(* Logix 5000 AddOnInstructionDefinition export I_1769scOF4IH; software revision 18.02 *)

TYPE STRING_32 :   // string type
STRUCT
   LEN : DINT;
   DATA : SINT[32];
END_STRUCT
END_TYPE

TYPE STRING_8 :   // string type
STRUCT
   LEN : DINT;
   DATA : SINT[8];
END_STRUCT
END_TYPE

TYPE P_EUTable :
STRUCT
   Code : DINT;   // Engineering Units Code Number
   Desc : STRING_8;   // Engineering Units Text
END_STRUCT
END_TYPE

TYPE HART_ChanData :   // Analog and HART Channel Data for one channel / device
STRUCT
   ModSts : SINT;   // I/O Module Status
   ChanSts : SINT;   // HART I/O Channel Status
   HARTSts : SINT;   // HART Device / Communication Status
   Initializing : BOOL;
   CommFail : BOOL;
   CurFault : BOOL;
   PassThruMSGAvail : BOOL;
   DataUpdateAvail : BOOL;
   BrokenWire : BOOL;
   StsUpdateAvail : BOOL;
   DeviceFault : BOOL;
   HARTCommErr : SINT;   // HART Communication Error Bits
   HARTCommErr0 : BOOL;
   BufferOverflow : BOOL;
   HARTCommErr2 : BOOL;
   ChecksumErr : BOOL;
   FramingErr : BOOL;
   OverrunErr : BOOL;
   ParityErr : BOOL;
   HasHARTCommErr : BOOL;
   HARTRespCode : SINT;   // HART Response Code
   HARTFieldDevSts : SINT;   // HART Field Device Status
   PVOutOfLimits : BOOL;
   VarOutOfLimits : BOOL;
   LoopCurSaturated : BOOL;
   LoopCurFixed : BOOL;
   Code48StsAvail : BOOL;
   ColdStart : BOOL;
   CfgChanged : BOOL;
   Malfunction : BOOL;
   HARTExtSts : SINT;   // HART Extended Status
   MaintReqd : BOOL;
   DeviceAlert : BOOL;
   PowerFail : BOOL;
   CalFault : BOOL;
   AV : REAL;   // Analog Value
   AVRawMin : REAL;   // Analog Signal Raw Range Minimum (here because it's not in DevInfo)
   AVRawMax : REAL;   // Analog Signal Raw Range Maximum (here because it's not in DevInfo)
   PV : REAL;   // HART Primary Variable
   SV : REAL;   // HART Secondary Variable
   TV : REAL;   // HART Tertiary Variable
   FV : REAL;   // HART Fourth Variable
   PVStatus : SINT;   // HART Primary Variable Status
   SVStatus : SINT;   // HART Secondary Variable Status
   TVStatus : SINT;   // HART Tertiary Variable Status
   FVStatus : SINT;   // HART Fourth Variable Status
   AVEU : STRING_8;   // Text for HART Range (Analog Value) Engineering Units
   PVEU : STRING_8;   // Text for HART PV Engineering Units
   SVEU : STRING_8;   // Text for HART SV Engineering Units
   TVEU : STRING_8;   // Text for HART TV Engineering Units
   FVEU : STRING_8;   // Text for HART FV Engineering Units
   Diag : SINT[28];   // Channel Diagnostic bit array (from HART Code 48 message)
   DevInfo : HART_DevInfo;   // HART Device Information
   Cfg_AutoUpdDevInfo : BOOL;   // 1=automatically update device info, 0=no auto update
   Cfg_ManUpdDevInfo : BOOL;   // 1=allow manual device info update request, 0=disallow
   MCmd_UpdDevInfo : BOOL;   // Maintenance Command to request update of device info
END_STRUCT
END_TYPE

TYPE STRING_16 :   // string type
STRUCT
   LEN : DINT;
   DATA : SINT[16];
END_STRUCT
END_TYPE

TYPE HART_DevInfo :   // HART Device Information for one channel / device
STRUCT
   CmdSts : SINT;   // HART Command Status Success=0
   MfrID : SINT;   // Manufacturer ID
   DevType : SINT;   // Device Type
   Preamble : SINT;   // HART Preamble
   UnivCmdCode : SINT;   // Universal Command Code
   XducerSpecRev : SINT;   // Transducer Specification Revision
   SwRev : SINT;   // Software Revision Number
   HwRev : SINT;   // Hardware Revision Number
   HARTFlags : SINT;   // HART Flags
   pad9 : SINT;
   MfrID_16 : INT;   // 16-bit Manufacturer ID
   DevID : DINT;   // Device ID Number (serial number)
   Tag : STRING_8;   // Tag String
   Desc : STRING_16;   // Descriptor String
   DateDay : SINT;   // Device Revision Date: Day of the Month
   DateMonth : SINT;   // Device Revision Date: Month of the Year
   DateYear : INT;   // Device Revision Date: Year
   FinalAssyNum : DINT;   // Final Assembly Number
   Message : STRING_32;   // Message String
   PVCode : SINT;   // Primary Variable Identifier
   SVCode : SINT;   // Secondary Variable Identifier
   TVCode : SINT;   // Third Variable Identifier
   FVCode : SINT;   // Fourth Variable Identifier
   PVUnits : SINT;   // Primary Variable Units of Measure (enum)
   SVUnits : SINT;   // Secondary Variable Units of Measure (enum)
   TVUnits : SINT;   // Third Variable Units of Measure (enum)
   FVUnits : SINT;   // Fourth Variable Units of Measure (enum)
   XferFunc : SINT;   // Transfer Function
   RangeUnits : SINT;   // Analog Value Range Units of Measure
   ExpDevType : INT;   // Expanded Device Type Code
   AVRangeMin : REAL;   // Analog Value in Engineering Units at 4.00 mADC
   AVRangeMax : REAL;   // Analog Value in Engineering Units at 20.00 mADC
   DampVal : REAL;   // Damping Value
   WriteProtCode : SINT;   // Write Protect Code
   pad117 : SINT;
   PrivLblMfr : INT;   // Private Label Manufacturer ID
END_STRUCT
END_TYPE

ADD_ON_INSTRUCTION I_1769scOF4IH   (* revision 3.5 01 Release, vendor Rockwell Automation *)
// Spectrum Controls 1769sc-OF4IH
// HART Isolated AO Module
// Revision note:
// See V3.5-xx Release Notes for details. New Instruction for V3.5 of Library of Premier Integration Objects.
// Help:
// Copyright © Rockwell Automation, Inc.  All Rights Reserved.
// This instruction provides 4 analog outputs for one 1769sc-OF4IH
// HART Isolated Analog output module.  It reads the input and
// configuration assemblies from the module and copies the data into
// individual structures for each of the four output channels. The
// instruction also uses a MSG instruction to read updated Device
// Information (DevInfo) for each channel.  These structures are then
// used by the P_AOutHART instruction to provide channel data,
// device configuration and diagnostic information for each individual
// HART device.
VAR_IN_OUT
   Ref_Inp : SC:1769sc_OF4IH:I:0; {required}   // HART Module Input assembly for the 1769sc-OF4IH. e.g. Local:1:I
   Ref_Cfg : SC:1769sc_OF4IH:C:0; {required}   // HART Module Config assembly for the 1769sc-OF4IH. e.g. Local:1:C
   Ref_Out : SC:1769sc_OF4IH:O:0; {required}   // HART Module Output assembly for the 1769sc-OF4IH. e.g. Local:1:O
END_VAR
VAR_INPUT
   Inp_IOFault : BOOL; {visible}   // I/O Communication Fail (from GSV)
END_VAR
VAR_IN_OUT
   Ref_ChanData : HART_ChanData[4]; {required}   // HART Channel Data for each of 4 Channels
   Ref_EUTable : P_EUTable[1]; {required}
END_VAR
VAR_OUTPUT
   I_1769scOF4IH : BOOL;   // Unique Parameter Name for auto - discovery
END_VAR
VAR
   Wrk_Chan : DINT; {access None}   // Channel Number (pointer) for DevInfo copy
   Wrk_InpDINT : DINT; {access None}   // Bit pattern of REAL input
   Wrk_Packet : DINT; {access None}   // Packet Number being received in Input Assembly
   Wrk_ChanPrev : DINT; {access None}   // Channel value last scan
   Wrk_PktPrev : DINT; {access None}   // Packet value last scan
   Wrk_NewHARTData : BOOL; {access None}   // New packet of HART data received in I/O scan
   Wrk_EUTextFSC : CONTROL := (LEN := 1); {access None}   // Engineering units text lookup FSC
END_VAR

ROUTINE Logic   (* ladder *)
// Process Compact I/O 4-channel HART Isolated Analog Output module
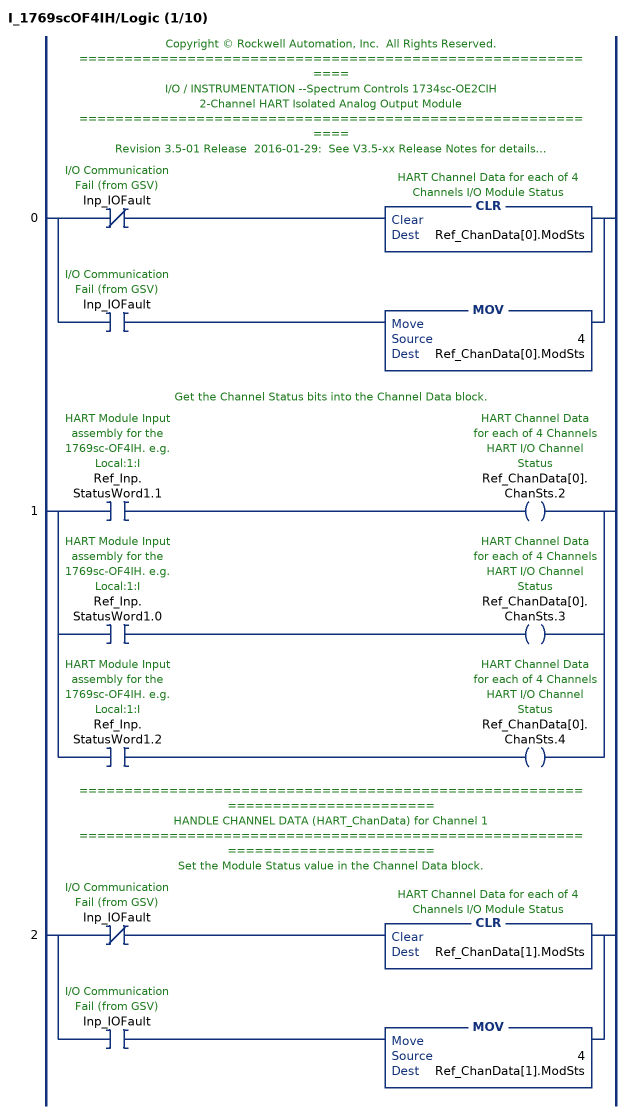
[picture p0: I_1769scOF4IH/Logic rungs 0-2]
   // Copyright © Rockwell Automation, Inc.  All Rights Reserved.
   // ============================================================
   // I/O / INSTRUMENTATION --Spectrum Controls 1734sc-OE2CIH
   // 2-Channel HART Isolated Analog Output Module
   // ============================================================
   // Revision 3.5-01 Release  2016-01-29:  See V3.5-xx Release Notes for details.
   // V3.5-01  2016-01-29:  New Instruction for V3.5 of Library of Premier Integration Objects.
   // ============================================================
   // This Instruction manages a Spectrum Controls Point I/O 2-channel
   // Isolated Analog Output Module with HART.
   // ============================================================
   // HANDLE CHANNEL DATA (HART_ChanData) for Channel 0
   // ============================================================
   // Set the Module Status value in the Channel Data block.
   0: [XIO(Inp_IOFault) CLR(Ref_ChanData[0].ModSts) ,XIC(Inp_IOFault) MOV(4,Ref_ChanData[0].ModSts) ];
   // Get the Channel Status bits into the Channel Data block.
   1: [XIC(Ref_Inp.StatusWord1.1) OTE(Ref_ChanData[0].ChanSts.2) ,XIC(Ref_Inp.StatusWord1.0) OTE(Ref_ChanData[0].ChanSts.3) ,XIC(Ref_Inp.StatusWord1.2) OTE(Ref_ChanData[0].ChanSts.4) ];
   // ===============================================================================
   // HANDLE CHANNEL DATA (HART_ChanData) for Channel 1
   // ===============================================================================
   // Set the Module Status value in the Channel Data block.
   2: [XIO(Inp_IOFault) CLR(Ref_ChanData[1].ModSts) ,XIC(Inp_IOFault) MOV(4,Ref_ChanData[1].ModSts) ];
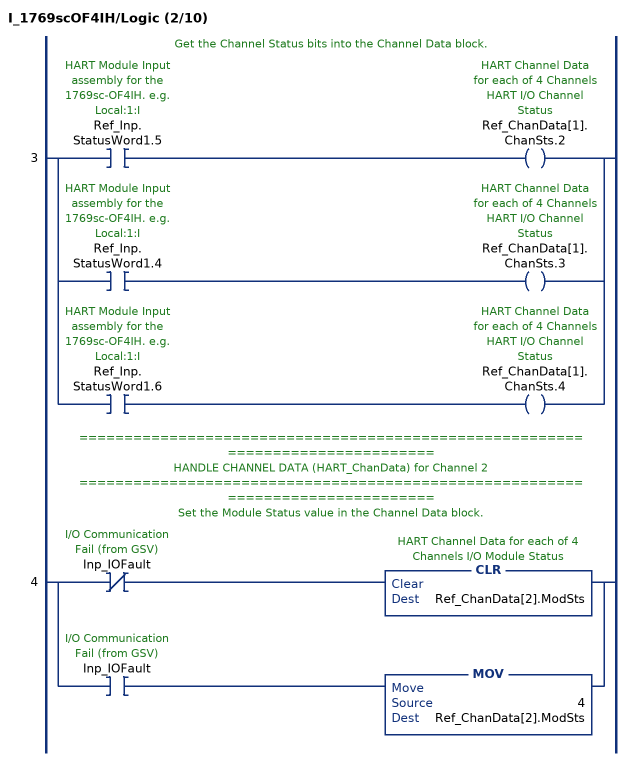
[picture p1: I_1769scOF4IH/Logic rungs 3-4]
   // Get the Channel Status bits into the Channel Data block.
   3: [XIC(Ref_Inp.StatusWord1.5) OTE(Ref_ChanData[1].ChanSts.2) ,XIC(Ref_Inp.StatusWord1.4) OTE(Ref_ChanData[1].ChanSts.3) ,XIC(Ref_Inp.StatusWord1.6) OTE(Ref_ChanData[1].ChanSts.4) ];
   // ===============================================================================
   // HANDLE CHANNEL DATA (HART_ChanData) for Channel 2
   // ===============================================================================
   // Set the Module Status value in the Channel Data block.
   4: [XIO(Inp_IOFault) CLR(Ref_ChanData[2].ModSts) ,XIC(Inp_IOFault) MOV(4,Ref_ChanData[2].ModSts) ];
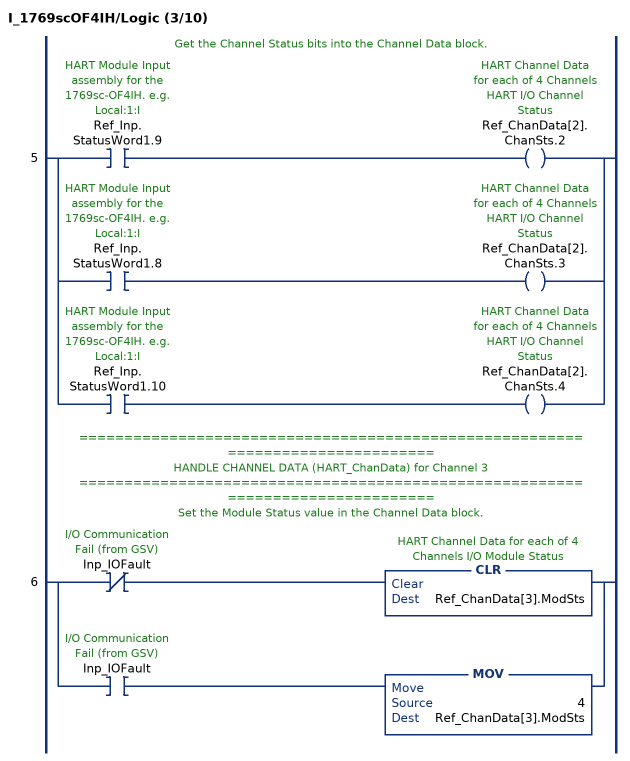
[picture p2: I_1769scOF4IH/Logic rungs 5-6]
   // Get the Channel Status bits into the Channel Data block.
   5: [XIC(Ref_Inp.StatusWord1.9) OTE(Ref_ChanData[2].ChanSts.2) ,XIC(Ref_Inp.StatusWord1.8) OTE(Ref_ChanData[2].ChanSts.3) ,XIC(Ref_Inp.StatusWord1.10) OTE(Ref_ChanData[2].ChanSts.4) ];
   // ===============================================================================
   // HANDLE CHANNEL DATA (HART_ChanData) for Channel 3
   // ===============================================================================
   // Set the Module Status value in the Channel Data block.
   6: [XIO(Inp_IOFault) CLR(Ref_ChanData[3].ModSts) ,XIC(Inp_IOFault) MOV(4,Ref_ChanData[3].ModSts) ];
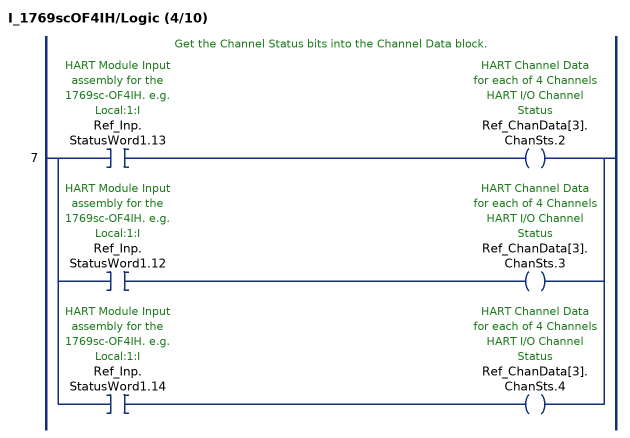
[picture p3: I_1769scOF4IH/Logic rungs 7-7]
   // Get the Channel Status bits into the Channel Data block.
   7: [XIC(Ref_Inp.StatusWord1.13) OTE(Ref_ChanData[3].ChanSts.2) ,XIC(Ref_Inp.StatusWord1.12) OTE(Ref_ChanData[3].ChanSts.3) ,XIC(Ref_Inp.StatusWord1.14) OTE(Ref_ChanData[3].ChanSts.4) ];
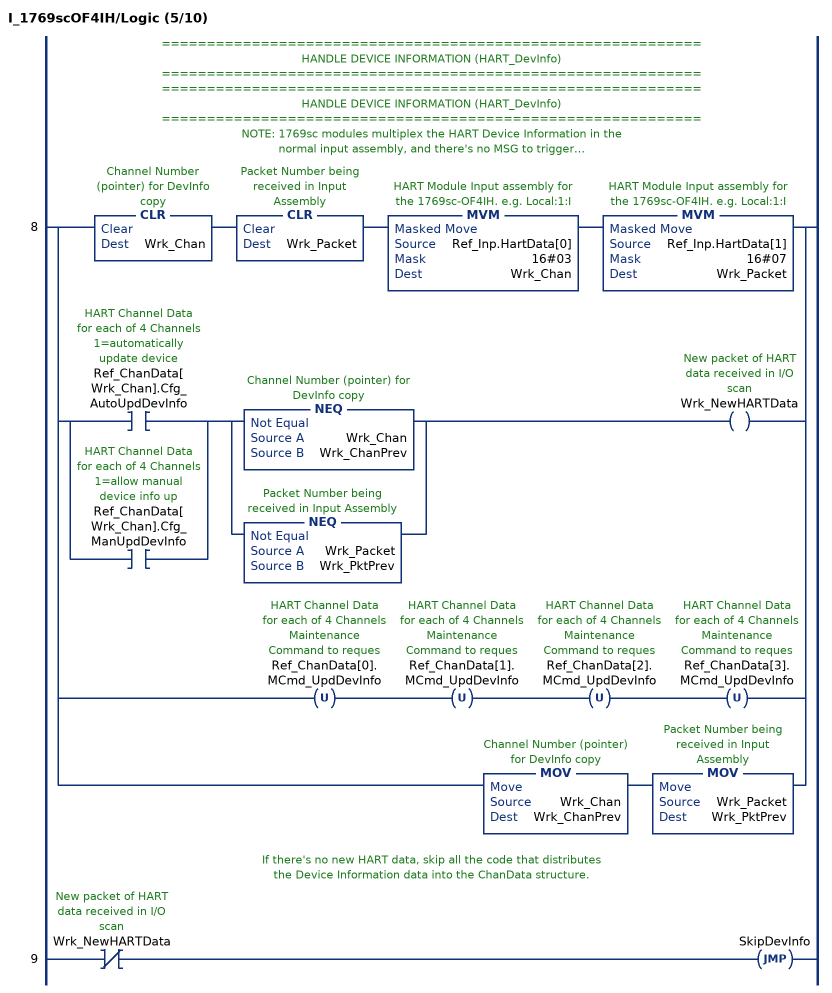
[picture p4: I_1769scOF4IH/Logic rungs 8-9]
   // ============================================================
   // HANDLE DEVICE INFORMATION (HART_DevInfo)
   // ============================================================
   // ============================================================
   // HANDLE DEVICE INFORMATION (HART_DevInfo)
   // ============================================================
   // NOTE: 1769sc modules multiplex the HART Device Information in the
   // normal input assembly, and there's no MSG to trigger.
   // If auto OR MANUAL update of Device Info is enabled,
   // update the information as received, and just clear any
   // command to refresh DevInfo (as command is not used).
   8: [CLR(Wrk_Chan) CLR(Wrk_Packet) MVM(Ref_Inp.HartData[0],16#03,Wrk_Chan) MVM(Ref_Inp.HartData[1],16#07,Wrk_Packet) ,[XIC(Ref_ChanData[Wrk_Chan].Cfg_AutoUpdDevInfo) ,XIC(Ref_ChanData[Wrk_Chan].Cfg_ManUpdDevInfo) ] [NEQ(Wrk_Chan,Wrk_ChanPrev) ,NEQ(Wrk_Packet,Wrk_PktPrev) ] OTE(Wrk_NewHARTData) ,OTU(Ref_ChanData[0].MCmd_UpdDevInfo) OTU(Ref_ChanData[1].MCmd_UpdDevInfo) OTU(Ref_ChanData[2].MCmd_UpdDevInfo) OTU(Ref_ChanData[3].MCmd_UpdDevInfo) ,MOV(Wrk_Chan,Wrk_ChanPrev) MOV(Wrk_Packet,Wrk_PktPrev) ];
   // If there's no new HART data, skip all the code that distributes
   // the Device Information data into the ChanData structure.
   9: XIO(Wrk_NewHARTData)JMP(SkipDevInfo);
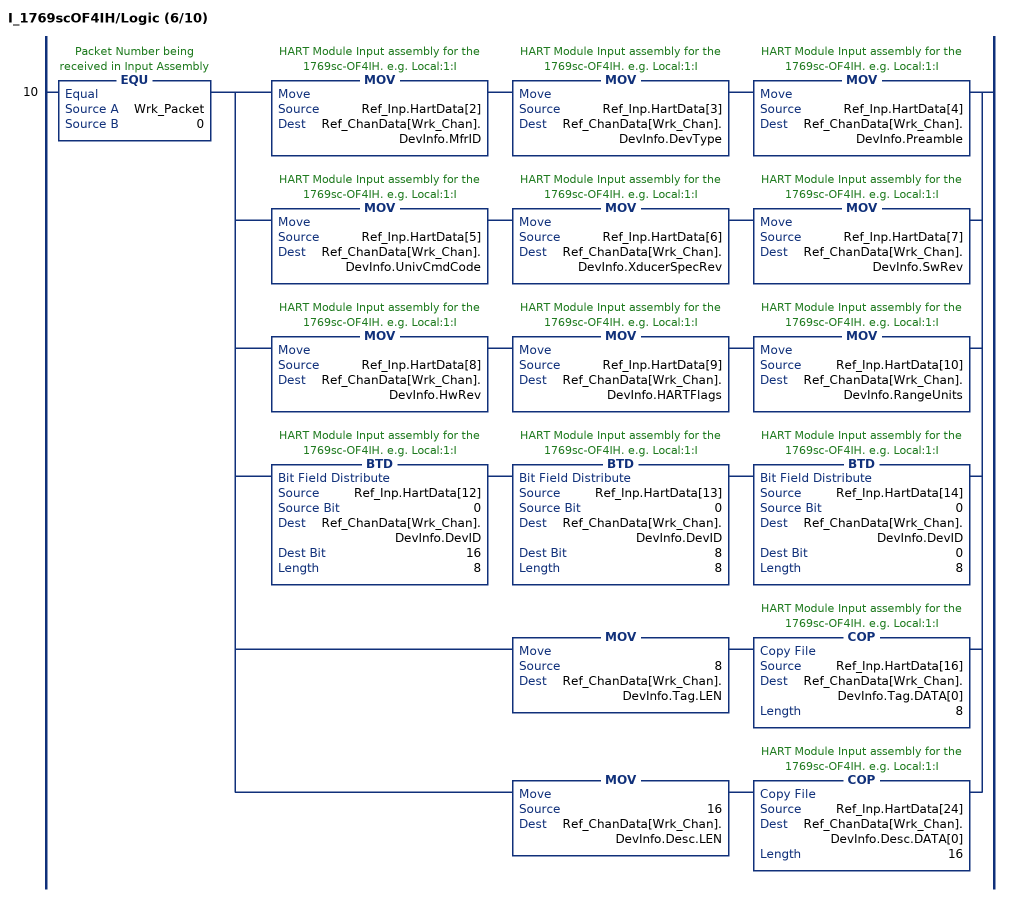
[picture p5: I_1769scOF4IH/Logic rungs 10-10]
   10: EQU(Wrk_Packet,0)[MOV(Ref_Inp.HartData[2],Ref_ChanData[Wrk_Chan].DevInfo.MfrID) MOV(Ref_Inp.HartData[3],Ref_ChanData[Wrk_Chan].DevInfo.DevType) MOV(Ref_Inp.HartData[4],Ref_ChanData[Wrk_Chan].DevInfo.Preamble) ,MOV(Ref_Inp.HartData[5],Ref_ChanData[Wrk_Chan].DevInfo.UnivCmdCode) MOV(Ref_Inp.HartData[6],Ref_ChanData[Wrk_Chan].DevInfo.XducerSpecRev) MOV(Ref_Inp.HartData[7],Ref_ChanData[Wrk_Chan].DevInfo.SwRev) ,MOV(Ref_Inp.HartData[8],Ref_ChanData[Wrk_Chan].DevInfo.HwRev) MOV(Ref_Inp.HartData[9],Ref_ChanData[Wrk_Chan].DevInfo.HARTFlags) MOV(Ref_Inp.HartData[10],Ref_ChanData[Wrk_Chan].DevInfo.RangeUnits) ,BTD(Ref_Inp.HartData[12],0,Ref_ChanData[Wrk_Chan].DevInfo.DevID,16,8) BTD(Ref_Inp.HartData[13],0,Ref_ChanData[Wrk_Chan].DevInfo.DevID,8,8) BTD(Ref_Inp.HartData[14],0,Ref_ChanData[Wrk_Chan].DevInfo.DevID,0,8) ,MOV(8,Ref_ChanData[Wrk_Chan].DevInfo.Tag.LEN) COP(Ref_Inp.HartData[16],Ref_ChanData[Wrk_Chan].DevInfo.Tag.DATA[0],8) ,MOV(16,Ref_ChanData[Wrk_Chan].DevInfo.Desc.LEN) COP(Ref_Inp.HartData[24],Ref_ChanData[Wrk_Chan].DevInfo.Desc.DATA[0],16) ];
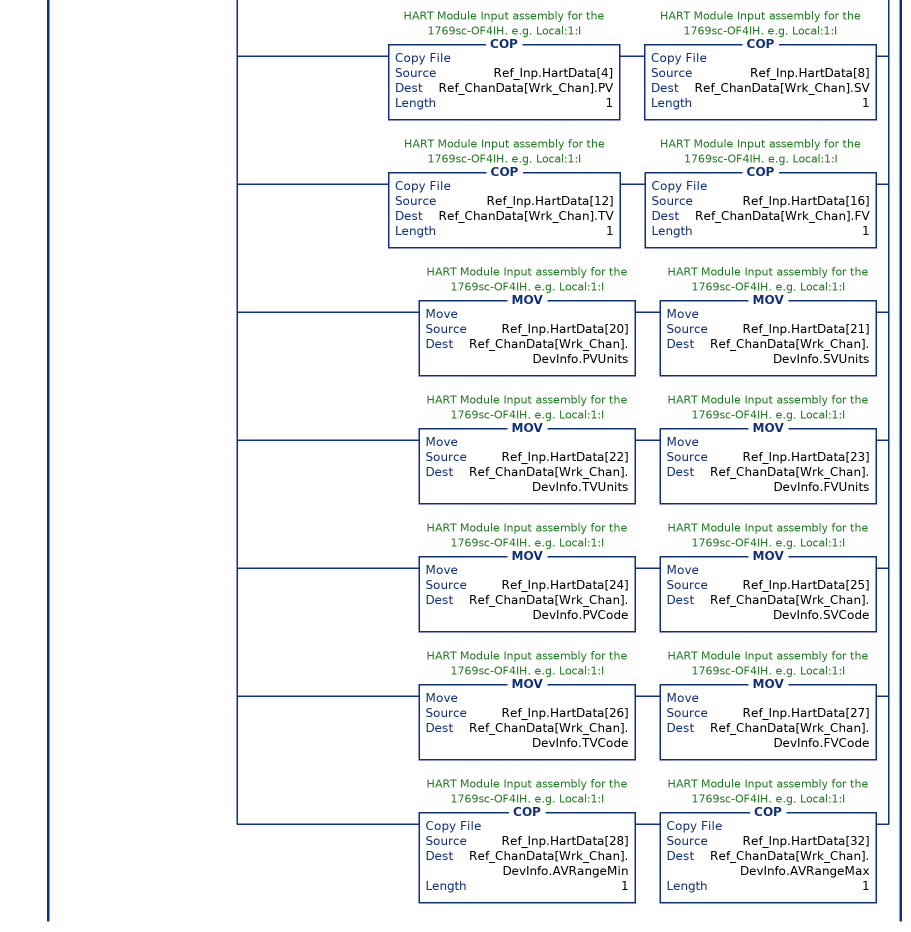
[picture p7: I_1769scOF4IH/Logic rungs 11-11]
   // Get the HART Communication Error bits, HART Response Code,
   // HART Field Device Status and HART Extended Status into the Channel Data block.
   11: EQU(Wrk_Packet,1)[XIC(Ref_Inp.HartData[2].7) [CLR(Ref_ChanData[Wrk_Chan].HARTRespCode) MOV(Ref_Inp.HartData[2],Ref_ChanData[Wrk_Chan].HARTCommErr) ,CLR(Ref_ChanData[Wrk_Chan].PVStatus) CLR(Ref_ChanData[Wrk_Chan].SVStatus) ,CLR(Ref_ChanData[Wrk_Chan].TVStatus) CLR(Ref_ChanData[Wrk_Chan].FVStatus) ] ,XIO(Ref_Inp.HartData[2].7) [MOV(Ref_Inp.HartData[2],Ref_ChanData[Wrk_Chan].HARTRespCode) CLR(Ref_ChanData[Wrk_Chan].HARTCommErr) ,MOV(-64,Ref_ChanData[Wrk_Chan].PVStatus) MOV(-64,Ref_ChanData[Wrk_Chan].SVStatus) ,MOV(-64,Ref_ChanData[Wrk_Chan].TVStatus) MOV(-64,Ref_ChanData[Wrk_Chan].FVStatus) ] ,MOV(Ref_Inp.HartData[3],Ref_ChanData[Wrk_Chan].HARTFieldDevSts) CLR(Ref_ChanData[Wrk_Chan].HARTExtSts) ,COP(Ref_Inp.HartData[4],Ref_ChanData[Wrk_Chan].PV,1) COP(Ref_Inp.HartData[8],Ref_ChanData[Wrk_Chan].SV,1) ,COP(Ref_Inp.HartData[12],Ref_ChanData[Wrk_Chan].TV,1) COP(Ref_Inp.HartData[16],Ref_ChanData[Wrk_Chan].FV,1) ,MOV(Ref_Inp.HartData[20],Ref_ChanData[Wrk_Chan].DevInfo.PVUnits) MOV(Ref_Inp.HartData[21],Ref_ChanData[Wrk_Chan].DevInfo.SVUnits) ,MOV(Ref_Inp.HartData[22],Ref_ChanData[Wrk_Chan].DevInfo.TVUnits) MOV(Ref_Inp.HartData[23],Ref_ChanData[Wrk_Chan].DevInfo.FVUnits) ,MOV(Ref_Inp.HartData[24],Ref_ChanData[Wrk_Chan].DevInfo.PVCode) MOV(Ref_Inp.HartData[25],Ref_ChanData[Wrk_Chan].DevInfo.SVCode) ,MOV(Ref_Inp.HartData[26],Ref_ChanData[Wrk_Chan].DevInfo.TVCode) MOV(Ref_Inp.HartData[27],Ref_ChanData[Wrk_Chan].DevInfo.FVCode) ,COP(Ref_Inp.HartData[28],Ref_ChanData[Wrk_Chan].DevInfo.AVRangeMin,1) COP(Ref_Inp.HartData[32],Ref_ChanData[Wrk_Chan].DevInfo.AVRangeMax,1) ];
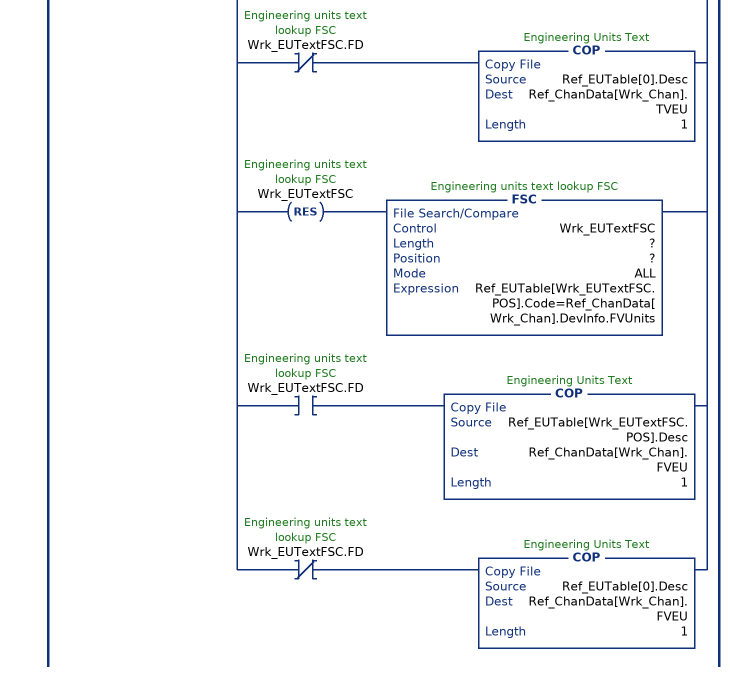
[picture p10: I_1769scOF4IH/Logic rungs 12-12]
   12: EQU(Wrk_Packet,1)[SIZE(Ref_EUTable,0,Wrk_EUTextFSC.LEN) ,RES(Wrk_EUTextFSC) FSC(Wrk_EUTextFSC,?,?,ALL,Ref_EUTable[Wrk_EUTextFSC.POS].Code=Ref_ChanData[Wrk_Chan].DevInfo.RangeUnits) ,XIC(Wrk_EUTextFSC.FD) COP(Ref_EUTable[Wrk_EUTextFSC.POS].Desc,Ref_ChanData[Wrk_Chan].AVEU,1) ,XIO(Wrk_EUTextFSC.FD) COP(Ref_EUTable[0].Desc,Ref_ChanData[Wrk_Chan].AVEU,1) ,RES(Wrk_EUTextFSC) FSC(Wrk_EUTextFSC,?,?,ALL,Ref_EUTable[Wrk_EUTextFSC.POS].Code=Ref_ChanData[Wrk_Chan].DevInfo.PVUnits) ,XIC(Wrk_EUTextFSC.FD) COP(Ref_EUTable[Wrk_EUTextFSC.POS].Desc,Ref_ChanData[Wrk_Chan].PVEU,1) ,XIO(Wrk_EUTextFSC.FD) COP(Ref_EUTable[0].Desc,Ref_ChanData[Wrk_Chan].PVEU,1) ,RES(Wrk_EUTextFSC) FSC(Wrk_EUTextFSC,?,?,ALL,Ref_EUTable[Wrk_EUTextFSC.POS].Code=Ref_ChanData[Wrk_Chan].DevInfo.SVUnits) ,XIC(Wrk_EUTextFSC.FD) COP(Ref_EUTable[Wrk_EUTextFSC.POS].Desc,Ref_ChanData[Wrk_Chan].SVEU,1) ,XIO(Wrk_EUTextFSC.FD) COP(Ref_EUTable[0].Desc,Ref_ChanData[Wrk_Chan].SVEU,1) ,RES(Wrk_EUTextFSC) FSC(Wrk_EUTextFSC,?,?,ALL,Ref_EUTable[Wrk_EUTextFSC.POS].Code=Ref_ChanData[Wrk_Chan].DevInfo.TVUnits) ,XIC(Wrk_EUTextFSC.FD) COP(Ref_EUTable[Wrk_EUTextFSC.POS].Desc,Ref_ChanData[Wrk_Chan].TVEU,1) ,XIO(Wrk_EUTextFSC.FD) COP(Ref_EUTable[0].Desc,Ref_ChanData[Wrk_Chan].TVEU,1) ,RES(Wrk_EUTextFSC) FSC(Wrk_EUTextFSC,?,?,ALL,Ref_EUTable[Wrk_EUTextFSC.POS].Code=Ref_ChanData[Wrk_Chan].DevInfo.FVUnits) ,XIC(Wrk_EUTextFSC.FD) COP(Ref_EUTable[Wrk_EUTextFSC.POS].Desc,Ref_ChanData[Wrk_Chan].FVEU,1) ,XIO(Wrk_EUTextFSC.FD) COP(Ref_EUTable[0].Desc,Ref_ChanData[Wrk_Chan].FVEU,1) ];
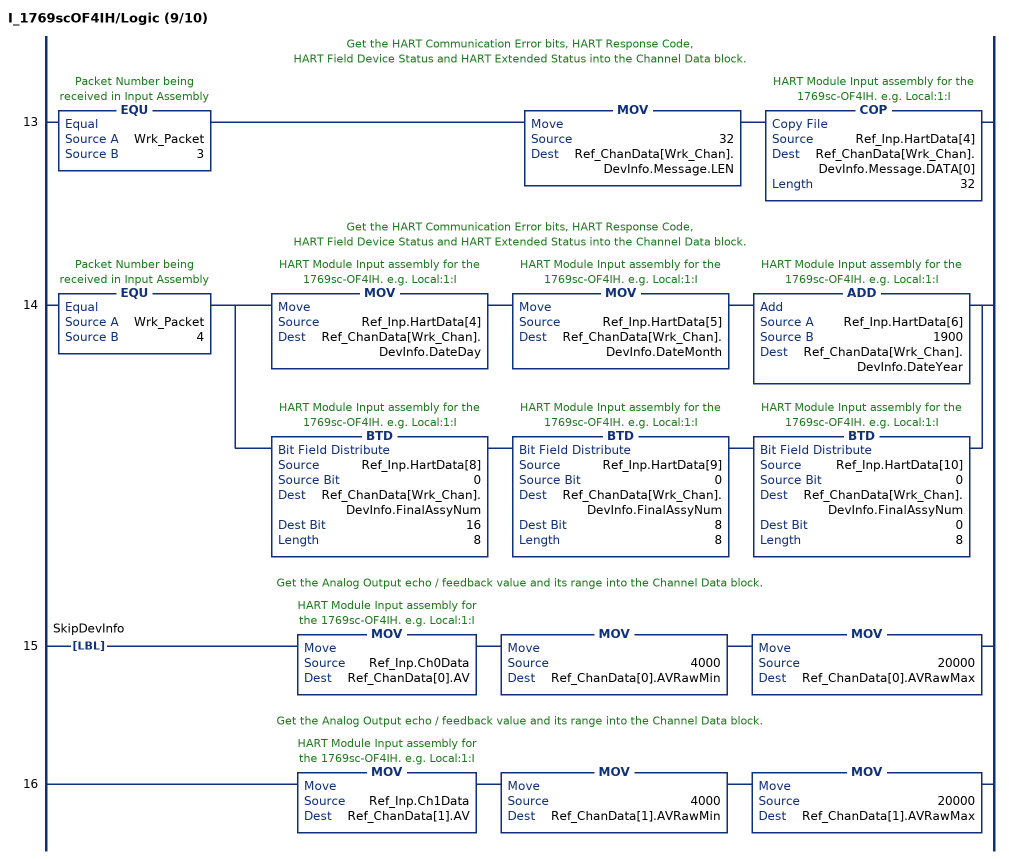
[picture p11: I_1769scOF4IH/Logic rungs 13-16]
   // Get the HART Communication Error bits, HART Response Code,
   // HART Field Device Status and HART Extended Status into the Channel Data block.
   13: EQU(Wrk_Packet,3)MOV(32,Ref_ChanData[Wrk_Chan].DevInfo.Message.LEN)COP(Ref_Inp.HartData[4],Ref_ChanData[Wrk_Chan].DevInfo.Message.DATA[0],32);
   // Get the HART Communication Error bits, HART Response Code,
   // HART Field Device Status and HART Extended Status into the Channel Data block.
   14: EQU(Wrk_Packet,4)[MOV(Ref_Inp.HartData[4],Ref_ChanData[Wrk_Chan].DevInfo.DateDay) MOV(Ref_Inp.HartData[5],Ref_ChanData[Wrk_Chan].DevInfo.DateMonth) ADD(Ref_Inp.HartData[6],1900,Ref_ChanData[Wrk_Chan].DevInfo.DateYear) ,BTD(Ref_Inp.HartData[8],0,Ref_ChanData[Wrk_Chan].DevInfo.FinalAssyNum,16,8) BTD(Ref_Inp.HartData[9],0,Ref_ChanData[Wrk_Chan].DevInfo.FinalAssyNum,8,8) BTD(Ref_Inp.HartData[10],0,Ref_ChanData[Wrk_Chan].DevInfo.FinalAssyNum,0,8) ];
   // Get the Analog Output echo / feedback value and its range into the Channel Data block.
   15: LBL(SkipDevInfo)MOV(Ref_Inp.Ch0Data,Ref_ChanData[0].AV)MOV(4000,Ref_ChanData[0].AVRawMin)MOV(20000,Ref_ChanData[0].AVRawMax);
   // Get the Analog Output echo / feedback value and its range into the Channel Data block.
   16: MOV(Ref_Inp.Ch1Data,Ref_ChanData[1].AV)MOV(4000,Ref_ChanData[1].AVRawMin)MOV(20000,Ref_ChanData[1].AVRawMax);
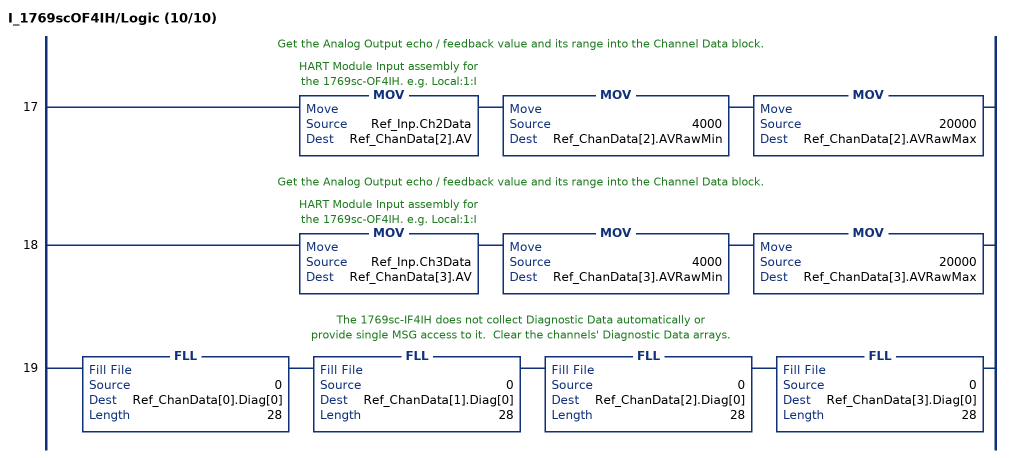
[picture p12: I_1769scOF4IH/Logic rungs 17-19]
   // Get the Analog Output echo / feedback value and its range into the Channel Data block.
   17: MOV(Ref_Inp.Ch2Data,Ref_ChanData[2].AV)MOV(4000,Ref_ChanData[2].AVRawMin)MOV(20000,Ref_ChanData[2].AVRawMax);
   // Get the Analog Output echo / feedback value and its range into the Channel Data block.
   18: MOV(Ref_Inp.Ch3Data,Ref_ChanData[3].AV)MOV(4000,Ref_ChanData[3].AVRawMin)MOV(20000,Ref_ChanData[3].AVRawMax);
   // The 1769sc-IF4IH does not collect Diagnostic Data automatically or
   // provide single MSG access to it.  Clear the channels' Diagnostic Data arrays.
   19: FLL(0,Ref_ChanData[0].Diag[0],28)FLL(0,Ref_ChanData[1].Diag[0],28)FLL(0,Ref_ChanData[2].Diag[0],28)FLL(0,Ref_ChanData[3].Diag[0],28);
END_ROUTINE
END_ADD_ON_INSTRUCTION
